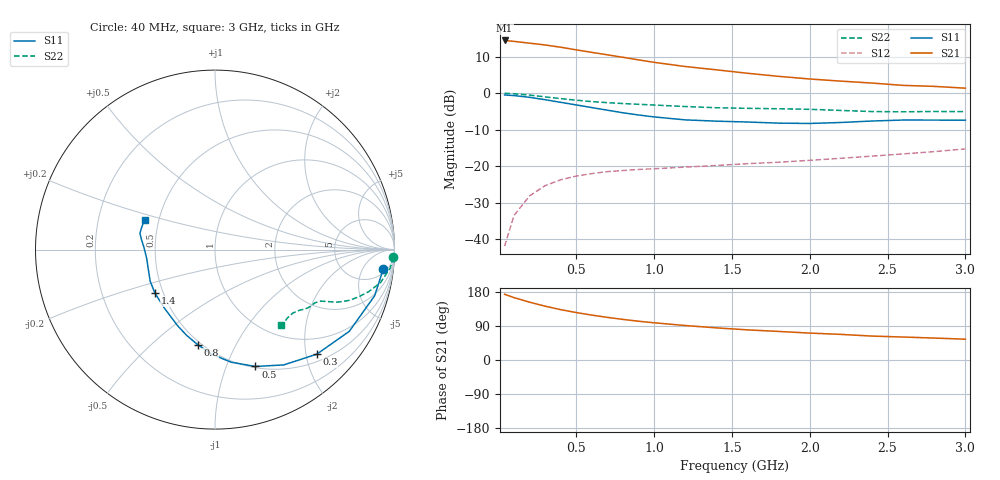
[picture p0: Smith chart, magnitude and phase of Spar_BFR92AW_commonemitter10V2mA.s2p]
! Filename:  BFR92AWF.S2P  Version:  4.0
! NXP part #: BFR92AW  Date: Jun 1994
! Bias condition: Vce=10V, Ic=2mA
#  MHz  S  MA  R  50
! Freq  S11  S21  S12  S22  !GUM [dB]
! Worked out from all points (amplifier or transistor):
!   21 points, 40 MHz to 3 GHz, reference 50 ohm
!   highest |S21| = 14.4 dB at 40 MHz (marker M1)
!   |S21| within 3 dB of that: start of sweep to 561.5 MHz
!   unconditionally stable (mu >= 1): 1.186 GHz to end of sweep
!   at 300 MHz: K = 0.32, MSG = 19.3 dB, |S12| = -25.4 dB
!   at 1 GHz: K = 0.86, MSG = 14.6 dB, |S12| = -20.7 dB
!   at 3 GHz: K = 1.28, MAG = 5.1 dB, |S12| = -15.3 dB
!   S11 on the Smith chart (normalised r, x): 40 MHz: 7, -14; 300 MHz: 0.64, -2.21; 500 MHz: 0.51, -1.27; 800 MHz: 0.48, -0.71; 1.4 GHz: 0.45, -0.26; 3 GHz: 0.42, +0.17
40  0.944 -6.5  5.268 173.4  0.008 86.2  0.995 -2.4
100  0.926 -16.1  5.117 164.7  0.021 79.9  0.981 -6.1
200  0.876 -31.3  4.836 152.6  0.039 70.2  0.94 -11.3
300  0.813 -45.8  4.571 142.1  0.054 62.8  0.888 -15.3
400  0.748 -59.2  4.255 132.9  0.065 57.6  0.841 -18.3
500  0.689 -70.9  3.915 125.2  0.073 53.8  0.8 -20.7
600  0.634 -81.8  3.618 118.5  0.079 51.7  0.766 -22.2
700  0.584 -91.6  3.35 112.5  0.084 50.3  0.74 -23.3
800  0.538 -100.4  3.097 107.1  0.087 49.7  0.72 -23.9
900  0.502 -108.6  2.855 102.3  0.09 49.3  0.703 -24.4
1000  0.472 -116.3  2.642 98.2  0.092 49.5  0.687 -24.9
1200  0.43 -131.4  2.315 91.0  0.097 50.7  0.655 -26.0
1400  0.413 -144.2  2.086 84.8  0.102 52.7  0.631 -28.0
1600  0.402 -153.9  1.871 79.5  0.108 55.5  0.619 -30.5
1800  0.388 -162.9  1.698 75.4  0.113 59.1  0.611 -32.1
2000  0.384 -173.1  1.562 71.0  0.12 62.3  0.6 -33.5
2200  0.396 178.2  1.46 67.6  0.128 65.3  0.579 -35.7
2400  0.415 171.8  1.374 63.1  0.137 67.9  0.559 -39.3
2600  0.428 167.7  1.277 60.6  0.147 70.5  0.555 -43.5
2800  0.427 163.1  1.237 57.9  0.158 73.3  0.56 -46.6
3000  0.426 157.2  1.169 54.9  0.172 75.4  0.558 -48.6
